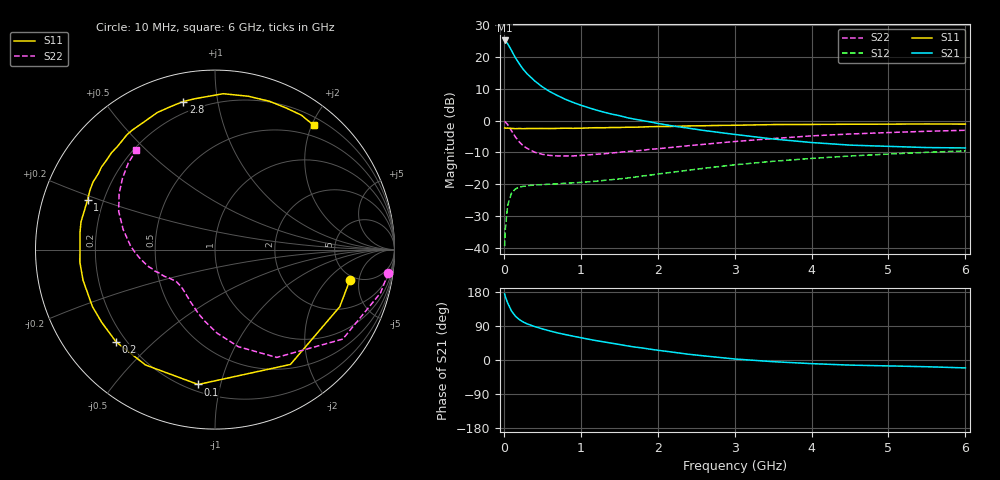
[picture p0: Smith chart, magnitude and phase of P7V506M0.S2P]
! SIEMENS Small Signal Semiconductors
! BFP196
! Si NPN RF Bipolar Junction Transistor in SOT143
! VCE = 0.5 V  IC = 6 mA
! Common Emitter S-Parameters:  May  1996
# GHz  S  MA  R  50
!  f  S11  S21  S12  S22
! GHz  MAG  ANG  MAG  ANG  MAG  ANG  MAG  ANG
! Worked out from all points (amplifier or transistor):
!   36 points, 10 MHz to 6 GHz, reference 50 ohm
!   highest |S21| = 25.3 dB at 10 MHz (marker M1)
!   |S21| within 3 dB of that: start of sweep to 96.11 MHz
!   unconditionally stable (mu >= 1): 963.8 MHz to end of sweep
!   at 250 MHz: K = 0.30, MSG = 18.5 dB, |S12| = -20.7 dB
!   at 1.4 GHz: K = 1.19, MAG = 7.7 dB, |S12| = -18.6 dB
!   at 6 GHz: K = 1.06, MAG = -1.1 dB, |S12| = -9.5 dB
!   S11 on the Smith chart (normalised r, x): 10 MHz: 4.53, -3.75; 100 MHz: 0.24, -0.85; 200 MHz: 0.16, -0.39; 1 GHz: 0.14, +0.18; 2.8 GHz: 0.14, +0.80; 6 GHz: 0.32, +2.03
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0.01  0.7707 -12.6  18.35 174.5  0.0106 84.9  0.9742 -7.7
0.02  0.7645 -24.6  17.83 167.0  0.0201 79.5  0.9531 -14.7
0.05  0.7655 -56.7  16.29 150.2  0.0469 62.0  0.8692 -35.0
0.1  0.7573 -97.1  12.74 129.3  0.0723 44.2  0.6922 -60.2
0.15  0.7505 -121.1  9.828 115.8  0.0842 34.1  0.5562 -76.5
0.2  0.7537 -136.9  7.919 106.9  0.09 28.1  0.4659 -88.5
0.25  0.7503 -147.3  6.486 100.4  0.0926 24.3  0.4052 -97.7
0.3  0.7531 -155.1  5.521 95.7  0.0949 22.3  0.3686 -104.5
0.4  0.7547 -166.9  4.25 88.2  0.0972 19.7  0.3197 -115.6
0.5  0.7561 -174.6  3.413 82.2  0.0986 18.9  0.2958 -123.3
0.6  0.7524 178.5  2.866 76.6  0.1004 19.0  0.2843 -128.8
0.7  0.7582 172.6  2.482 71.4  0.1015 19.3  0.2793 -133.2
0.8  0.7625 168.2  2.174 67.1  0.1039 20.1  0.2788 -136.8
1  0.7623 158.7  1.756 58.9  0.1069 22.2  0.2842 -142.4
1.1  0.7708 154.8  1.604 54.9  0.1094 23.1  0.29 -144.6
1.6  0.7897 137.0  1.12 37.4  0.1252 28.2  0.3271 -154.4
2.2  0.8141 118.9  0.826 20.6  0.1551 30.7  0.3824 -165.7
2.8  0.8438 102.1  0.654 6.8  0.1901 28.7  0.4482 -178.5
3.5  0.8697 87.0  0.516 -4.4  0.2299 22.5  0.5242 167.6
4.5  0.8804 69.8  0.413 -13.5  0.2784 11.9  0.6182 149.8
5.5  0.8904 57.3  0.378 -17.8  0.3183 1.0  0.6823 135.1
6  0.8844 51.6  0.373 -20.9  0.3349 -5.0  0.7075 128.2
